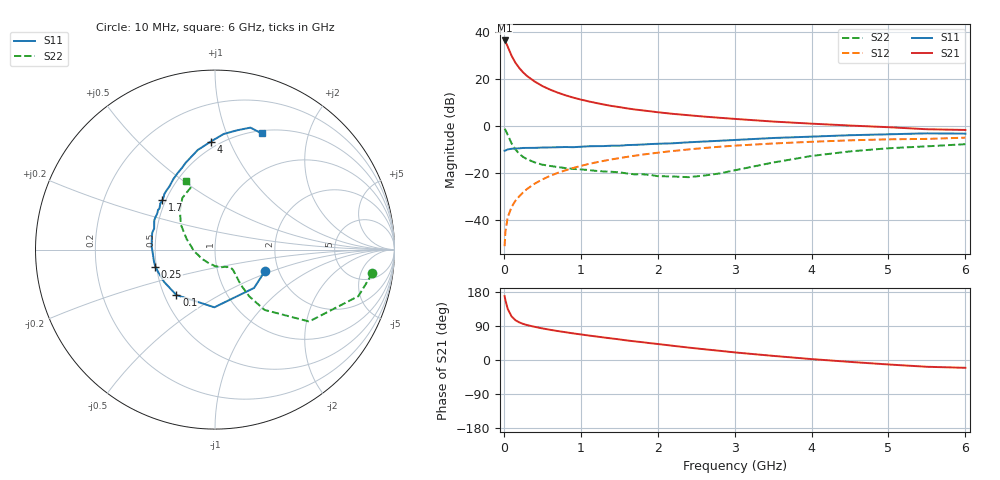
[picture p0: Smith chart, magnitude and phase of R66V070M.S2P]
! SIEMENS Small Signal Semiconductors
! BFR193
! Si NPN RF Bipolar Junction Transistor in SOT23
! VCE = 6 V  IC = 70 mA
! Common Emitter S-Parameters:  May  1996
# GHz  S  MA  R  50
!  f  S11  S21  S12  S22
! GHz  MAG  ANG  MAG  ANG  MAG  ANG  MAG  ANG
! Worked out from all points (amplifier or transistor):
!   36 points, 10 MHz to 6 GHz, reference 50 ohm
!   highest |S21| = 36.6 dB at 10 MHz (marker M1)
!   |S21| within 3 dB of that: start of sweep to 55.02 MHz
!   unconditionally stable (mu >= 1): 358.9 MHz to 2.069 GHz
!   at 250 MHz: K = 0.97, MSG = 25.6 dB, |S12| = -28.2 dB
!   at 1.4 GHz: K = 1.02, MAG = 10.5 dB, |S12| = -14.1 dB
!   at 6 GHz: K = 0.95, MSG = 1.6 dB, |S12| = -4.8 dB
!   S11 on the Smith chart (normalised r, x): 10 MHz: 1.70, -0.45; 100 MHz: 0.58, -0.33; 250 MHz: 0.49, -0.11; 1.7 GHz: 0.48, +0.31; 4 GHz: 0.45, +0.85; 6 GHz: 0.53, +1.34
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0.01  0.3031 -23.4  67.34 168.6  0.0028 80.2  0.8866 -8.6
0.02  0.3049 -44.5  63.92 158.3  0.0056 77.6  0.8397 -18.0
0.05  0.3215 -90.6  49.84 135.0  0.0115 70.0  0.6598 -37.4
0.1  0.3322 -130.4  31.96 115.2  0.019 68.6  0.4348 -50.6
0.15  0.336 -147.8  22.64 105.1  0.0259 70.0  0.3219 -53.8
0.2  0.3398 -157.8  17.46 99.3  0.0322 72.6  0.2615 -53.8
0.25  0.3459 -164.2  14.1 95.3  0.039 73.5  0.2228 -53.0
0.3  0.3464 -169.5  11.84 92.2  0.0461 74.9  0.2 -51.8
0.4  0.3474 -176.7  9.005 87.6  0.0599 74.9  0.1706 -49.9
0.5  0.353 177.5  7.21 83.4  0.0736 74.8  0.1524 -48.5
0.6  0.3555 172.5  6.051 79.8  0.0881 74.1  0.1431 -48.4
0.7  0.3583 169.0  5.219 76.4  0.1017 73.1  0.1361 -49.0
0.8  0.3622 164.9  4.581 73.4  0.1153 71.8  0.1289 -50.3
1.1  0.3754 154.3  3.399 64.7  0.1573 68.0  0.1174 -56.3
1.4  0.3863 145.2  2.714 56.9  0.1971 63.8  0.1075 -64.9
1.7  0.4021 137.0  2.285 49.2  0.2362 59.4  0.0947 -77.8
2.2  0.4349 125.6  1.839 37.5  0.2984 51.7  0.0852 -110.2
3.5  0.5634 99.8  1.263 10.9  0.4303 31.2  0.1691 159.4
4  0.6025 92.2  1.138 2.4  0.4684 24.2  0.2336 144.1
4.5  0.646 85.7  1.038 -5.0  0.5025 17.1  0.2922 132.1
5.5  0.7078 73.8  0.865 -17.9  0.5392 3.5  0.3744 110.5
6  0.6973 68.1  0.836 -20.6  0.5727 -0.4  0.4162 112.8
